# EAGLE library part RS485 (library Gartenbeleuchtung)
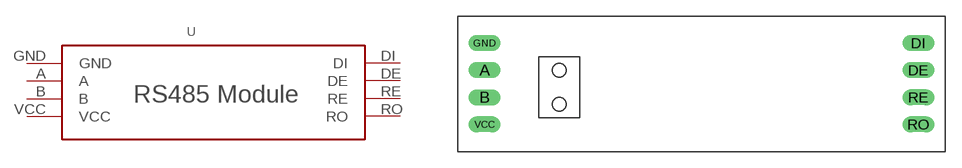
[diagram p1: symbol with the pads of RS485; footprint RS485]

Designator prefix -

## RS485  [RS485]
A  A
B  B
DE  DE
DI  DI
GND  GND  pwr
RE  RE
RO  RO
VCC  VCC  pwr

## Footprint RS485 (pad centres in mm)
drill 1 pad 1.422 long: A -20.32,0; B -20.32,-2.54; DE 20.32,0; DI 20.32,2.54; GND -20.32,2.54; RE 20.32,-2.54; RO 20.32,-5.08; VCC -20.32,-5.08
